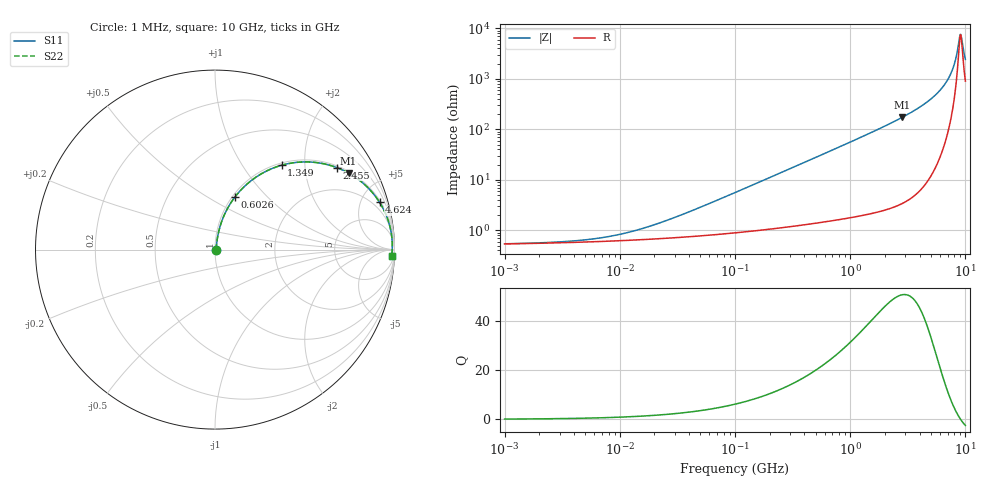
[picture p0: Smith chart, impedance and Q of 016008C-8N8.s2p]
# MHz S MA R 50
!Freq  MagS11  AngS11  MagS21  AngS21  MagS12  AngS12  MagS22  AngS22
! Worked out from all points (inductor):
!   801 points, 1 MHz to 10 GHz, reference 50 ohm
!   read as one part in series: L = 8.8 nH near 41.21 MHz
!   highest Q = 50.9 at 2.818 GHz (marker M1), where L = 9.74 nH
!   self-resonance near 9.016 GHz
!   S11 on the Smith chart (normalised r, x): 1 MHz: 1.01, +0.00; 602.6 MHz: 1.03, +0.67; 1.349 GHz: 1.04, +1.53; 2.455 GHz: 1.06, +2.93; 4.624 GHz: 1.18, +6.90; 10 GHz: 19, -45
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1  0.005392 5.8  0.9946 -0.0  0.9946 -0.0  0.005392 5.8
4.677351  0.006359 23.7  0.9942 -0.1  0.9942 -0.1  0.006359 23.7
10.11579  0.008335 41.5  0.9938 -0.3  0.9938 -0.3  0.008335 41.5
21.62719  0.01368 59.6  0.9931 -0.7  0.9931 -0.7  0.01368 59.6
101.1579  0.05606 77.7  0.9896 -3.2  0.9896 -3.2  0.05606 77.7
231.7395  0.1263 77.9  0.9813 -7.2  0.9813 -7.2  0.1263 77.9
467.7351  0.2482 72.7  0.9558 -14.4  0.9558 -14.4  0.2482 72.7
602.5596  0.3135 69.2  0.9359 -18.3  0.9359 -18.3  0.3135 69.2
912.0108  0.4481 61.5  0.8791 -26.6  0.8791 -26.6  0.4481 61.5
1348.963  0.599 51.7  0.785 -36.8  0.785 -36.8  0.599 51.7
2162.719  0.7773 37.8  0.613 -51.0  0.613 -51.0  0.7773 37.8
2454.709  0.8183 34.0  0.5586 -54.9  0.5586 -54.9  0.8183 34.0
2818.383  0.8579 29.8  0.4973 -59.1  0.4973 -59.1  0.8579 29.8
4623.81  0.954 16.0  0.2762 -72.5  0.2762 -72.5  0.954 16.0
5956.621  0.9779 9.7  0.1691 -77.7  0.1691 -77.7  0.9779 9.7
7161.434  0.9864 5.4  0.09451 -79.0  0.09451 -79.0  0.9864 5.4
7943.282  0.9881 3.0  0.05383 -75.7  0.05383 -75.7  0.9881 3.0
8317.638  0.9882 2.0  0.03639 -70.0  0.03639 -70.0  0.9882 2.0
8709.636  0.9878 0.9  0.02042 -52.9  0.02042 -52.9  0.9878 0.9
9015.711  0.9873 0.2  0.01304 -12.9  0.01304 -12.9  0.9873 0.2
9332.543  0.9865 -0.6  0.01708 37.7  0.01708 37.7  0.9865 -0.6
10000  0.9843 -2.2  0.04046 66.1  0.04046 66.1  0.9843 -2.2
